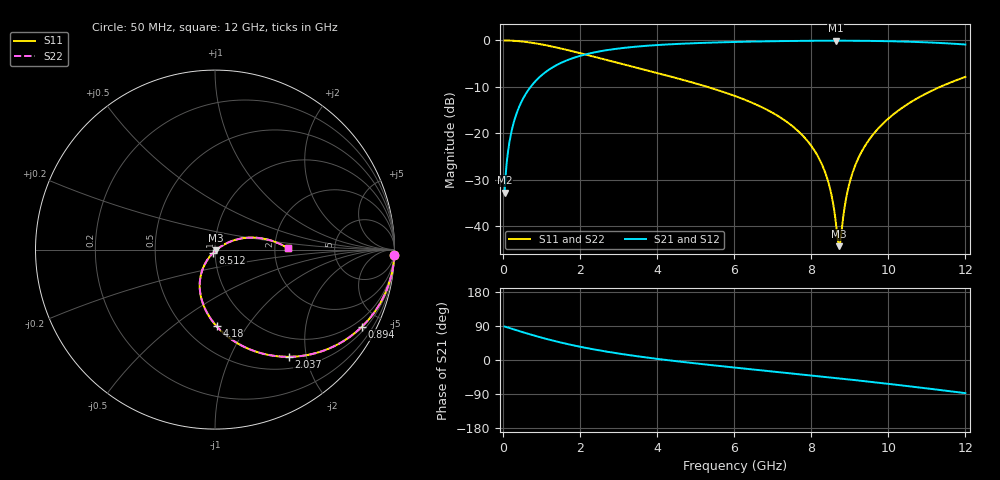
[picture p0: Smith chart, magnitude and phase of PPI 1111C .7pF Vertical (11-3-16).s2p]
# GHz S MA R 50
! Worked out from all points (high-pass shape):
!   1601 points, 50 MHz to 12 GHz, reference 50 ohm
!   highest |S21| = -0.06 dB at 8.639 GHz (marker M1); lowest = -32.8 dB at 50 MHz (marker M2)
!   |S21| within 3 dB of the highest: 2.125 GHz to end of sweep
!   lowest |S11| = -44.3 dB at 8.729 GHz (marker M3), VSWR 1.01, Z = 50.4 - j0.455 ohm
!   |S11| at or under -10 dB: 5.306 GHz to 11.35 GHz (6.04 GHz wide, 72.5 % of centre)
!   |S22| runs from -44.3 to 0.0 dB; largest |S21 - S12| = 0
!   S11 on the Smith chart (normalised r, x): 50 MHz: 1, -71; 894 MHz: 0.67, -3.95; 2.037 GHz: 0.67, -1.69; 4.18 GHz: 0.70, -0.73; 8.512 GHz: 0.98, -0.04; 12 GHz: 2.36, +0.05
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0.05  0.9997 -1.6  0.02296 88.4  0.02296 88.4  0.9997 -1.6
0.1769688  0.9967 -5.7  0.08103 84.3  0.08103 84.3  0.9967 -5.7
0.3263437  0.9889 -10.5  0.1483 79.5  0.1483 79.5  0.9889 -10.5
0.5653438  0.9677 -17.9  0.2516 72.0  0.2516 72.0  0.9677 -17.9
0.8939687  0.9245 -27.7  0.3806 62.3  0.3806 62.3  0.9245 -27.7
2.036688  0.7244 -55.6  0.6877 34.3  0.6877 34.3  0.7244 -55.6
2.044156  0.7231 -55.7  0.6891 34.2  0.6891 34.2  0.7231 -55.7
2.97775  0.5749 -72.3  0.8159 17.5  0.8159 17.5  0.5749 -72.3
4.038312  0.4424 -87.1  0.8939 2.6  0.8939 2.6  0.4424 -87.1
4.180219  0.4269 -88.8  0.9012 0.8  0.9012 0.8  0.4269 -88.8
6.025  0.252 -109.2  0.9634 -20.1  0.9634 -20.1  0.252 -109.2
7.249875  0.1435 -121.0  0.9844 -32.9  0.9844 -32.9  0.1435 -121.0
8.019156  0.07163 -126.6  0.9916 -41.0  0.9916 -41.0  0.07163 -126.6
8.310438  0.04312 -126.5  0.9929 -44.1  0.9929 -44.1  0.04312 -126.5
8.512094  0.02312 -121.5  0.9934 -46.2  0.9934 -46.2  0.02312 -121.5
8.639062  0.01105 -104.8  0.9935 -47.6  0.9935 -47.6  0.01105 -104.8
8.728687  0.006072 -48.0  0.9935 -48.6  0.9935 -48.6  0.006072 -48.0
8.95275  0.02466 24.2  0.993 -51.0  0.993 -51.0  0.02466 24.2
9.161875  0.04707 28.7  0.992 -53.4  0.992 -53.4  0.04707 28.7
9.512906  0.08638 28.2  0.989 -57.3  0.989 -57.3  0.08638 28.2
10.01331  0.1453 24.0  0.9816 -63.1  0.9816 -63.1  0.1453 24.0
12  0.4044 1.2  0.9046 -87.4  0.9046 -87.4  0.4044 1.2
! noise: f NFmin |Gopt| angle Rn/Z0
0.05  0.001241  0.9773  1.529  0.01247
1.372  0.00484  0.7505  12.13  0.003867
2.701  0.007891  0.7004  18.92  0.005022
4.031  0.0107  0.678  25.83  0.006112
5.36  0.01346  0.6688  32.61  0.007216
6.682  0.01625  0.6685  39.11  0.008406
8.012  0.01922  0.675  45.35  0.009773
9.341  0.02244  0.6869  51.28  0.0114
10.67  0.02602  0.7032  56.89  0.01341
12  0.0301  0.7232  62.22  0.01596
